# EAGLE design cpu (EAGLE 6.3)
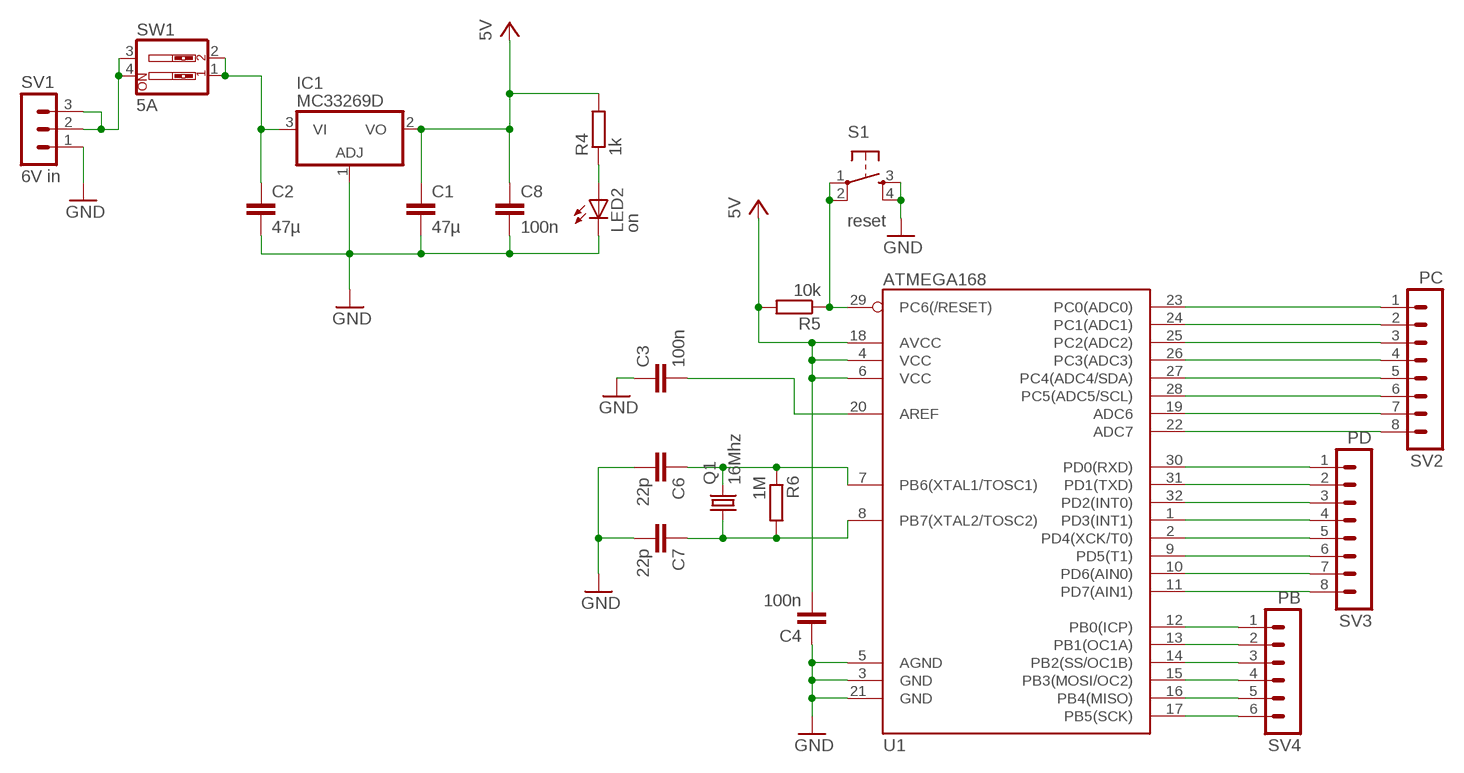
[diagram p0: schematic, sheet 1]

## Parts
C1  47µ  C2.5/5  [C2.5-5]
C2  47µ  C2.5/5  [C2.5-5]
C3  100n  C2.5/5  [C2.5-5]
C4  100n  C2.5/5  [C2.5-5]
C6  22p  C2.5/5  [C2.5-5]
C7  22p  C2.5/5  [C2.5-5]
C8  100n  C2.5/5  [C2.5-5]
IC1  MC33269D  [DPACK]
LED2  on  LED5MM  [LED5MM]
Q1  16Mhz  CRYSTALHC49U-V  [HC49U-V]
R4  1k  R-EU_0207/10  [0207/10]
R5  10k  R-EU_0207/10  [0207/10]
R6  1M  R-EU_0207/10  [0207/10]
S1  reset  TAC_SWITCHSMD  [TACTILE_SWITCH_SMD]
SV1  6V in  MA03-1  [MA03-1]
SV2  PC  MA08-1  [MA08-1]
SV3  PD  MA08-1  [MA08-1]
SV4  PB  MA06-1  [MA06-1]
SW1  5A  SW_DIP-2  [EDG-02]
U1  ATMEGA168  [TQFP32-08]

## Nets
GND: C1.2 C2.2 C3.1 C4.1 C6.2 C7.2 C8.2 IC1.1(ADJ) LED2.K(C) S1.3 S1.4 SV1.1 U1.3(GND) U1.5(AGND) U1.21(GND)
N$1: C2.1 IC1.3(VI) SW1.1 SW1.2
N$2: R5.1 S1.1 S1.2 U1.29(PC6(/RESET))
N$3: C3.2 U1.20(AREF)
N$4: C6.1 Q1.2 R6.1 U1.7(PB6(XTAL1/TOSC1))
N$5: C7.1 Q1.1 R6.2 U1.8(PB7(XTAL2/TOSC2))
N$6: LED2.A R4.1
N$7: SV2.1 U1.23(PC0(ADC0))
N$8: SV1.2 SV1.3 SW1.3 SW1.4
N$9: SV2.2 U1.24(PC1(ADC1))
N$10: SV2.3 U1.25(PC2(ADC2))
N$11: SV2.4 U1.26(PC3(ADC3))
N$12: SV2.5 U1.27(PC4(ADC4/SDA))
N$13: SV2.6 U1.28(PC5(ADC5/SCL))
N$14: SV2.7 U1.19(ADC6)
N$15: SV2.8 U1.22(ADC7)
N$16: SV3.1 U1.30(PD0(RXD))
N$17: SV3.2 U1.31(PD1(TXD))
N$18: SV3.3 U1.32(PD2(INT0))
N$19: SV3.4 U1.1(PD3(INT1))
N$20: SV3.5 U1.2(PD4(XCK/T0))
N$21: SV3.6 U1.9(PD5(T1))
N$22: SV3.7 U1.10(PD6(AIN0))
N$23: SV3.8 U1.11(PD7(AIN1))
N$24: SV4.1 U1.12(PB0(ICP))
N$25: SV4.2 U1.13(PB1(OC1A))
N$26: SV4.3 U1.14(PB2(SS/OC1B))
N$27: SV4.4 U1.15(PB3(MOSI/OC2))
N$28: SV4.5 U1.16(PB4(MISO))
N$29: SV4.6 U1.17(PB5(SCK))
VCC: C1.1 C4.2 C8.1 IC1.2(VO) R4.2 R5.2 U1.4(VCC) U1.6(VCC) U1.18(AVCC) ; supply symbol labelled 5V

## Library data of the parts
C1-C4 C6-C8 = capacitor-wima:C: CAPACITOR
IC1 = linear:MC33269?*: Adjustable Output Low Dropout Voltage Regulator 800 mA Source: http://www.onsemi.com/pub/Collateral/MC33269-D.PDF
LED2 = led:LED: LED
Q1 = crystal:CRYSTAL: CRYSTAL; OC_FARNELL: 1666969; OC_NEWARK: unknown
R4-R6 = rcl:R-EU_: RESISTOR, European symbol
S1 = SparkFun:TAC_SWITCH: Momentary Switch Button commonly used for reset or general input. Spark Fun Electronics SKU : COM-00097
SV1 = con-lstb:MA03-1: PIN HEADER; OC_FARNELL: unknown; OC_NEWARK: unknown
SV2 SV3 = con-lstb:MA08-1: PIN HEADER; OC_FARNELL: unknown; OC_NEWARK: unknown
SV4 = con-lstb:MA06-1: PIN HEADER; OC_FARNELL: unknown; OC_NEWARK: unknown
SW1 = special:SW_DIP-2: DIP SWITCH
U1 = SparkFun:ATMEGA168

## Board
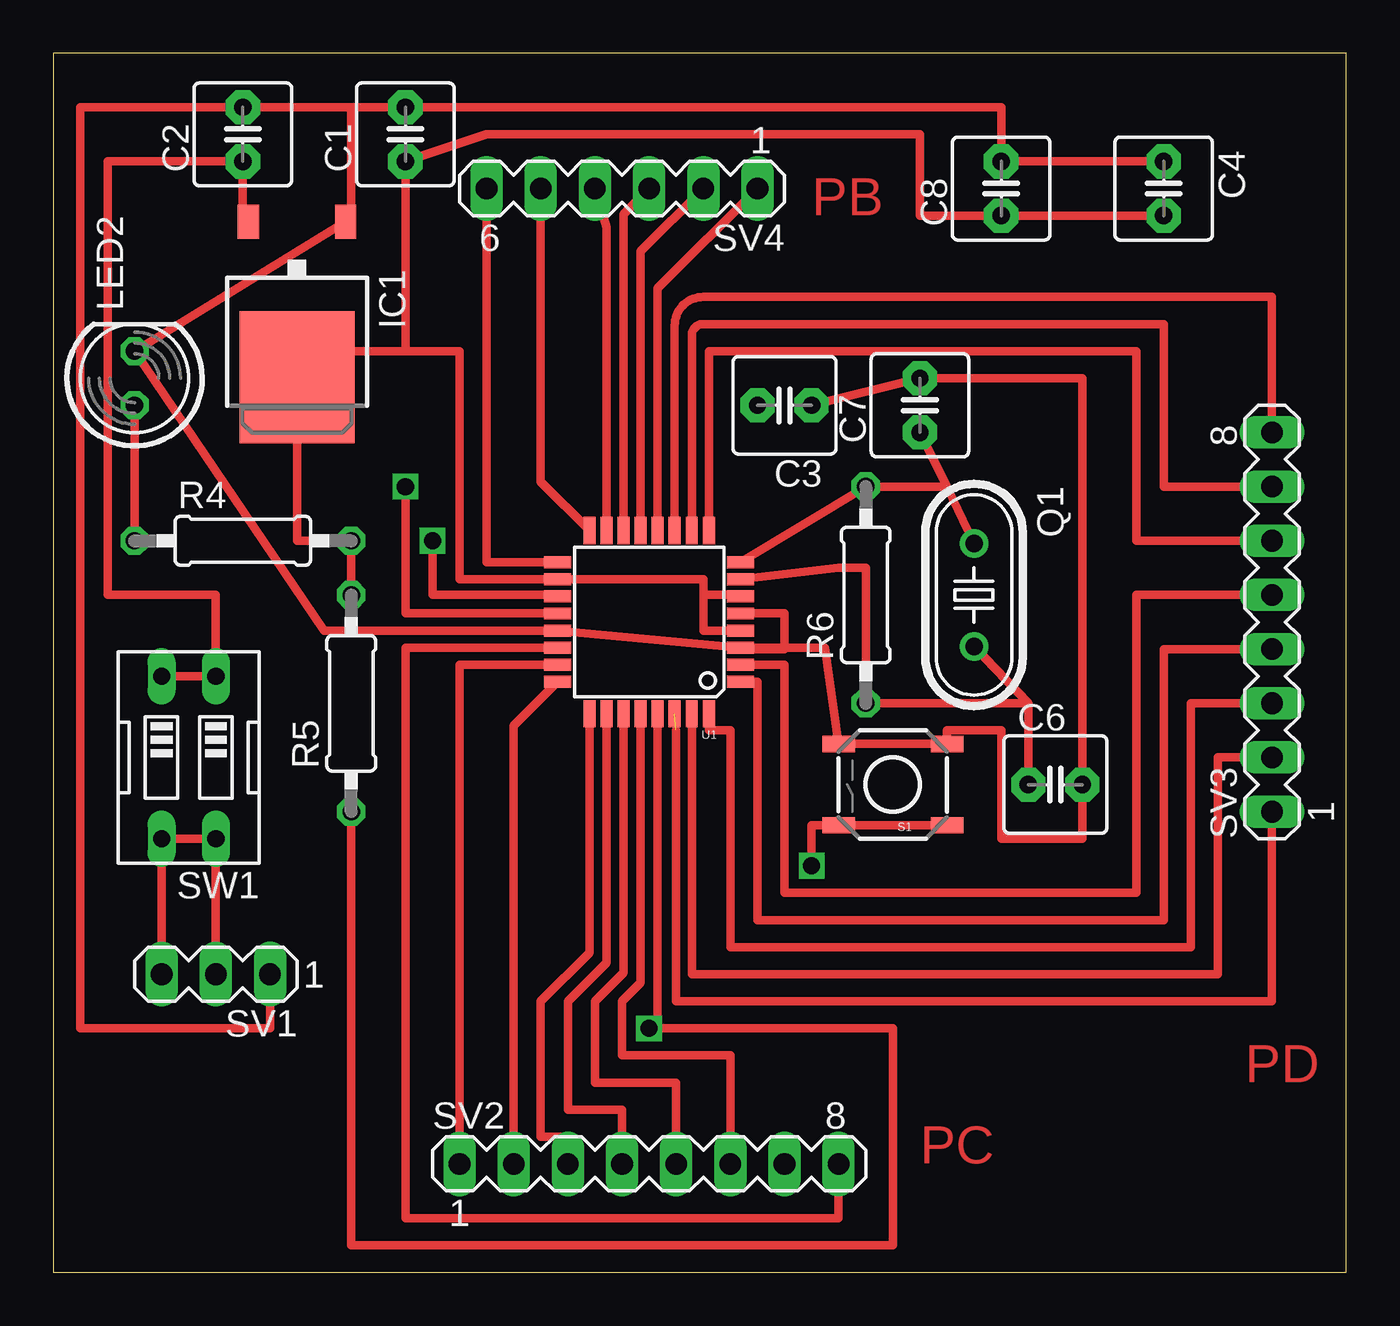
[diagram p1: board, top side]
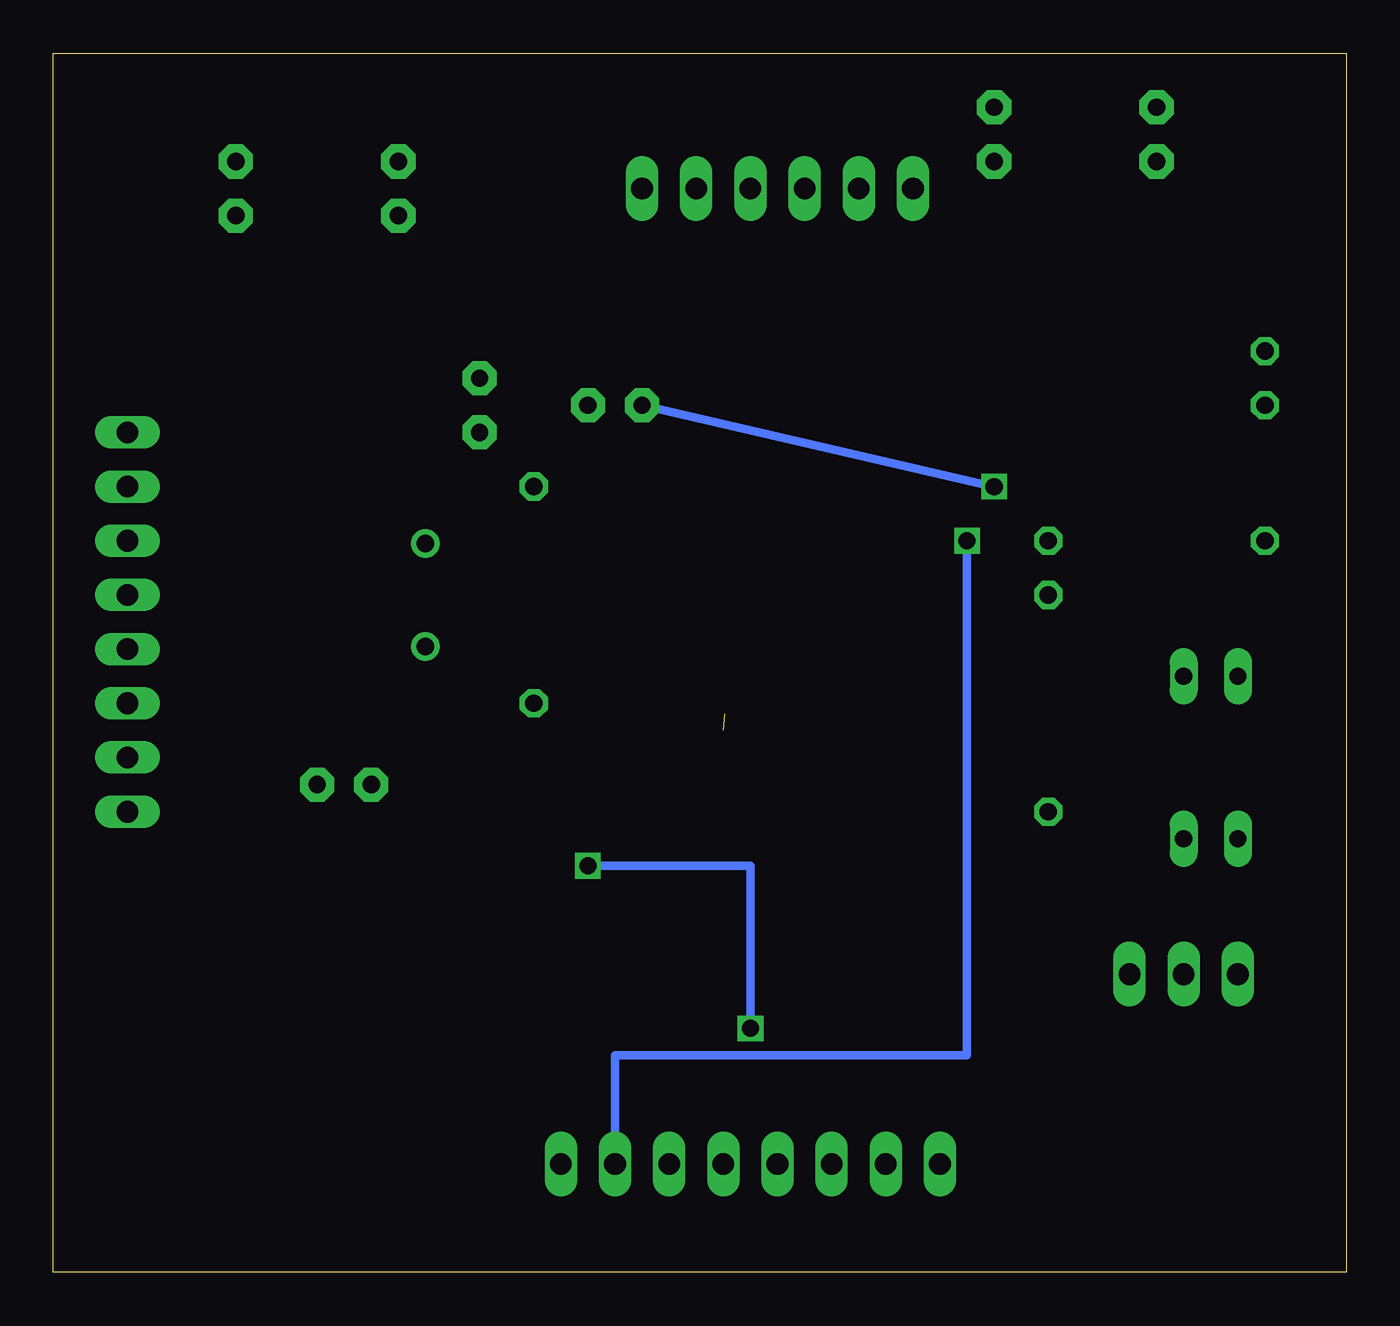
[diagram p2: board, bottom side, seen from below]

Size 60.63 x 57.14 mm. Coordinates in mm from the lower left corner, seen from the top.
Outline: 0,0 60.63,0 60.63,57.14 0,57.14 0,0
Copper layers (1*16): Top 0.035mm / dielectric 1.5mm / Bottom 0.035mm
Design rules "default": minimum track width 10mil, minimum drill 24mil, track to track 8mil, track to pad 8mil, pad to pad 8mil, via to via 8mil, smd to smd 8mil, copper to edge 40mil, drill to drill 8mil, minimum pad ring 10mil, minimum via ring 8mil, stop-mask expansion 4mil, vias tented up to drill 0mil, thermal gap 10mil

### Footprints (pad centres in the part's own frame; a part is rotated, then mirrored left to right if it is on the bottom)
C2.5-5 = drill 0.813 pad 1.6 octagon: 1 -1.27,0; 2 1.27,0
DPACK = smd 1 x 1.6: 1 -2.28,-4.8; 3 2.28,-4.8 | smd 5.4 x 6.2: 2 0,2.5
LED5MM = drill 0.813 octagon: A -1.27,0; K 1.27,0
HC49U-V = drill 0.813: 1 -2.413,0; 2 2.413,0
0207/10 = drill 0.813 octagon: 1 -5.08,0; 2 5.08,0
TACTILE_SWITCH_SMD = smd 1.524 x 0.762: 1 -2.54,1.905; 2 2.54,1.905; 3 -2.54,-1.905; 4 2.54,-1.905
MA03-1 = drill 1.016 long: 1 -2.54,0; 2 0,0; 3 2.54,0
MA08-1 = drill 1.016 long: 1 -8.89,0; 2 -6.35,0; 3 -3.81,0; 4 -1.27,0; 5 1.27,0; 6 3.81,0; 7 6.35,0; 8 8.89,0
MA06-1 = drill 1.016 long: 1 -6.35,0; 2 -3.81,0; 3 -1.27,0; 4 1.27,0; 5 3.81,0; 6 6.35,0
EDG-02 = drill 0.813 long: 1 -1.27,-3.81; 2 1.27,-3.81; 3 1.27,3.81; 4 -1.27,3.81
TQFP32-08 = smd 1.27 x 0.559: 1 -4.293,2.8; 2 -4.293,2; 3 -4.293,1.2; 4 -4.293,0.4; 5 -4.293,-0.4; 6 -4.293,-1.2; 7 -4.293,-2; 8 -4.293,-2.8; 17 4.293,-2.8; 18 4.293,-2; 19 4.293,-1.2; 20 4.293,-0.4; 21 4.293,0.4; 22 4.293,1.2; 23 4.293,2; 24 4.293,2.8 | smd 0.559 x 1.27: 9 -2.8,-4.293; 10 -2,-4.293; 11 -1.2,-4.293; 12 -0.4,-4.293; 13 0.4,-4.293; 14 1.2,-4.293; 15 2,-4.293; 16 2.8,-4.293; 25 2.8,4.293; 26 2,4.293; 27 1.2,4.293; 28 0.4,4.293; 29 -0.4,4.293; 30 -1.2,4.293; 31 -2,4.293; 32 -2.8,4.293

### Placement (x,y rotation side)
C1  16.51,53.34 90 top
C2  8.89,53.34 90 top
C3  34.29,40.64 180 top
C4  52.07,50.8 270 top
C6  46.99,22.86 0 top
C7  40.64,40.64 90 top
C8  44.45,50.8 90 top
IC1  11.43,44.45 180 top
LED2  3.81,41.91 90 top
Q1  43.18,31.75 270 top
R4  8.89,34.29 0 top
R5  13.97,26.67 90 top
R6  38.1,31.75 90 top
S1  39.37,22.86 180 top
SV1  7.62,13.97 180 top
SV2  27.94,5.08 0 top
SV3  57.15,30.48 90 top
SV4  26.67,50.8 180 top
SW1  6.35,24.13 180 top
U1  27.94,30.48 180 top

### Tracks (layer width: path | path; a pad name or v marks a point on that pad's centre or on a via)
GND
  Top 0.406: 13.97,54.61 C1.2 44.45,54.61 C8.2 C4.1 | 13.97,54.61 C2.2 1.27,54.61 1.27,11.43 10.16,11.43 SV1.1 | U1.3 U1.21 12.7,30.08 LED2.K IC1.1 13.97,49.25 13.97,54.61 | U1.5 34.29,30.88 34.29,29.21 32.23,29.21 U1.3 | U1.3 36.19,29.28 S1.4 S1.3 41.91,25.4 44.45,25.4 44.45,20.32 48.26,20.32 C6.2 48.26,41.91 C7.2 C3.1
N$1
  Top 0.406: SW1.2 SW1.1 7.62,31.75 2.54,31.75 2.54,52.07 C2.1 8.89,49.25 IC1.3
N$2  (via drill 0.8)
  Top 0.406: U1.29 28.34,11.83 v27.94,11.43 39.37,11.43 39.37,1.27 13.97,1.27 R5.1 | v35.56,19.05 35.56,20.95 S1.2 S1.1
  Bottom 0.406: v27.94,11.43 27.94,19.05 v35.56,19.05
N$3  (via drill 0.8)
  Top 0.406: U1.20 16.51,30.88 v16.51,36.83
  Bottom 0.406: v16.51,36.83 C3.2
N$4
  Top 0.406: 45.72,26.67 R6.1 38.1,33.02 36.83,33.02 U1.7 | 45.72,26.67 C6.1 | Q1.2 45.72,26.67
N$5
  Top 0.406: Q1.1 41.91,36.83 | 41.91,36.83 C7.1 | 41.91,36.83 R6.2 U1.8
N$6
  Top 0.406: R4.1 LED2.A
N$7
  Top 0.406: SV2.1 19.05,28.48 U1.23
N$8
  Top 0.406: SV1.3 SW1.3 SW1.4 SV1.2
N$9
  Top 0.406: SV2.2 21.59,25.62 U1.24
N$10
  Top 0.406: U1.25 25.14,14.98 22.86,12.7 22.86,6.35 24.13,6.35 SV2.3
N$11
  Top 0.406: U1.26 25.94,14.51 24.13,12.7 24.13,7.62 26.67,7.62 SV2.4
N$12
  Top 0.406: U1.27 26.74,14.04 25.4,12.7 25.4,8.89 29.21,8.89 SV2.5
N$13
  Top 0.406: U1.28 27.54,13.57 26.67,12.7 26.67,10.16 31.75,10.16 SV2.6
N$14  (via drill 0.8)
  Top 0.406: v17.78,34.29 17.78,31.75 23.65,31.75 U1.19
  Bottom 0.406: SV2.7 34.29,10.16 17.78,10.16 v17.78,34.29
N$15
  Top 0.406: SV2.8 36.83,2.54 16.51,2.54 16.51,29.28 U1.22
N$16  (1 unrouted)
  Top 0.406: SV3.1 57.15,12.7 29.21,12.7 29.21,25.4
N$17
  Top 0.406: SV3.2 54.61,24.13 54.61,13.97 29.94,13.97 U1.31
N$18
  Top 0.406: SV3.3 53.34,26.67 53.34,15.24 31.75,15.24 31.75,25.4 30.74,25.4 U1.32
N$19
  Top 0.406: U1.1 33.02,27.68 33.02,16.51 52.07,16.51 52.07,29.21 SV3.4
N$20
  Top 0.406: SV3.5 50.8,31.75 50.8,17.78 34.29,17.78 34.29,28.48 U1.2
N$21
  Top 0.406: SV3.6 50.8,34.29 50.8,43.18 30.74,43.18 U1.9
N$22
  Top 0.406: U1.10 29.94,43.91 arc-90 30.48,44.45 52.07,44.45 52.07,36.83 SV3.7
N$23
  Top 0.406: SV3.8 57.15,45.72 30.48,45.72 arc90 29.14,44.38 U1.11
N$24
  Top 0.406: SV4.1 28.34,46.12 U1.12
N$25
  Top 0.406: SV4.2 27.54,47.86 U1.13
N$26
  Top 0.406: SV4.3 26.74,49.6 U1.14
N$27
  Top 0.406: SV4.4 25.94,48.99 U1.15
N$28
  Top 0.406: U1.16 22.86,37.05 SV4.5
N$29
  Top 0.406: SV4.6 20.32,33.28 U1.17
VCC
  Top 0.406: C4.2 C8.1 40.64,49.53 40.64,53.34 20.32,53.34 C1.1 16.51,43.18 | U1.4 30.48,30.08 30.48,31.75 | 30.48,31.75 32.23,31.75 U1.6 | 30.48,31.75 30.48,32.48 U1.18 19.05,32.48 19.05,43.18 16.51,43.18 | 16.51,43.18 11.43,43.18 IC1.2 11.43,34.29 R4.2 R5.2

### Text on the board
Top: PB | PD | PC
